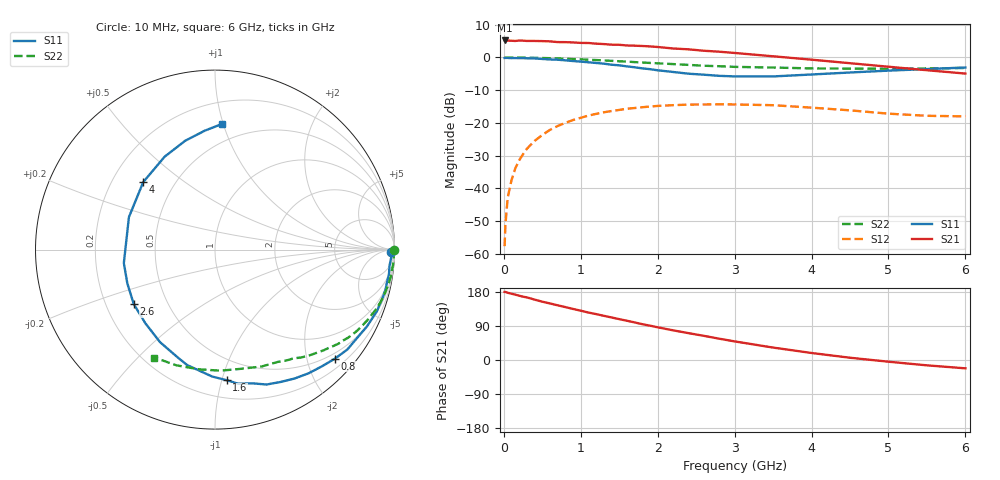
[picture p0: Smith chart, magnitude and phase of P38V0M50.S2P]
! SIEMENS Small Signal Semiconductors
! BFP181
! Si NPN RF Bipolar Junction Transistor in SOT143
! VCE = 8 V  IC = 0.5 mA
! Common Emitter S-Parameters:  March  1996
# GHz  S  MA  R  50
!  f  S11  S21  S12  S22
! GHz  MAG  ANG  MAG  ANG  MAG  ANG  MAG  ANG
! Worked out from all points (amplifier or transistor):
!   36 points, 10 MHz to 6 GHz, reference 50 ohm
!   highest |S21| = 5.2 dB at 10 MHz (marker M1)
!   |S21| within 3 dB of that: start of sweep to 2.533 GHz
!   unconditionally stable (mu >= 1): 3.827 GHz to end of sweep
!   at 250 MHz: K = 0.07, MSG = 17.4 dB, |S12| = -29.6 dB
!   at 1.4 GHz: K = 0.42, MSG = 10.2 dB, |S12| = -16.4 dB
!   at 6 GHz: K = 1.42, MAG = 2.7 dB, |S12| = -18.0 dB
!   S11 on the Smith chart (normalised r, x): 10 MHz: 75, -50; 800 MHz: 0.38, -2.54; 1.6 GHz: 0.33, -1.04; 2.6 GHz: 0.32, -0.28; 4 GHz: 0.33, +0.36; 6 GHz: 0.36, +0.99
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0.01  0.9817 -0.7  1.82 179.7  0.0013 86.6  0.9989 -0.1
0.02  0.9846 -1.1  1.805 179.6  0.0027 89.5  0.9986 -0.5
0.05  0.9835 -2.3  1.811 177.5  0.0072 87.3  0.9972 -1.3
0.1  0.9764 -5.4  1.801 174.9  0.0133 85.8  0.9969 -2.6
0.15  0.9788 -8.0  1.789 172.4  0.0203 83.2  0.9961 -3.9
0.2  0.9752 -10.5  1.816 169.6  0.0268 83.0  0.9949 -5.2
0.3  0.9716 -16.0  1.79 165.2  0.0402 78.8  0.992 -7.8
0.4  0.9647 -21.0  1.788 159.3  0.0529 75.0  0.988 -10.3
0.6  0.9322 -31.9  1.763 149.2  0.0781 67.2  0.9746 -15.5
0.8  0.9036 -42.2  1.715 139.6  0.1 59.9  0.9575 -20.2
1.1  0.8437 -58.4  1.664 125.2  0.1292 49.4  0.9239 -27.2
1.5  0.7577 -80.3  1.563 107.8  0.1576 36.8  0.8741 -35.5
1.6  0.7305 -84.9  1.525 103.6  0.1642 34.3  0.865 -37.3
1.9  0.6621 -103.5  1.476 90.6  0.1775 25.7  0.8249 -42.9
2.2  0.5998 -120.7  1.372 78.3  0.1864 18.3  0.7921 -47.9
2.6  0.5451 -146.1  1.267 63.8  0.191 9.6  0.7471 -54.2
3  0.5134 -171.6  1.172 49.1  0.1911 1.0  0.718 -60.5
3.5  0.5126 159.3  1.042 32.8  0.1862 -7.5  0.7011 -68.3
4  0.5491 136.7  0.925 18.5  0.1708 -13.9  0.6802 -77.4
4.5  0.589 118.4  0.817 6.0  0.1553 -18.4  0.6754 -87.4
5.5  0.6647 95.0  0.638 -14.1  0.1282 -16.3  0.6796 -108.4
6  0.7023 86.6  0.567 -22.0  0.1255 -12.4  0.6899 -119.3
